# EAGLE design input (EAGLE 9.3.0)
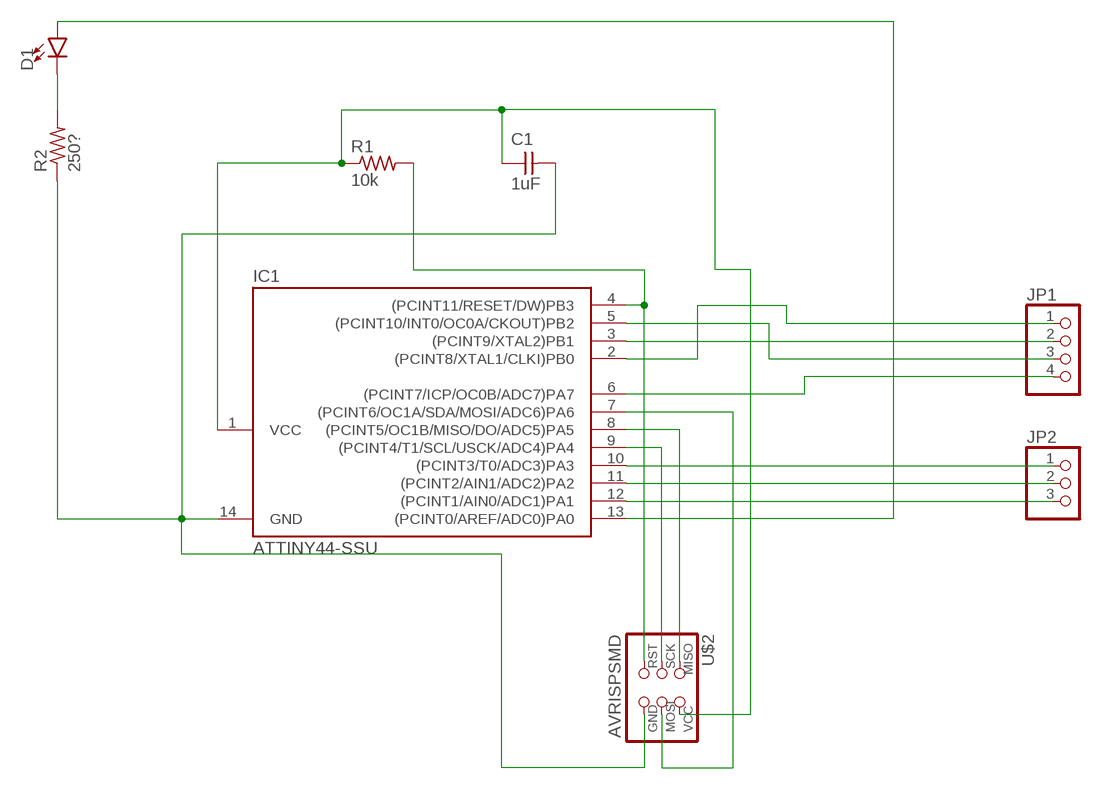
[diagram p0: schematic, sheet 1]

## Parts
C1  1uF  CAP-UNPOLARIZEDFAB  [C1206FAB]
D1  LED1206  [LED-1206]
IC1  ATTINY44-SSU  [SOIC14]
JP1  PINHD-1X41X04_SMT  [1X04_SMT]
JP2  PINHD-1X31X03_SMT  [1X03_SMT]
R1  10k  RES-US1206FAB  [R1206FAB]
R2  250?  RES-US1206FAB  [R1206FAB]
U$2  AVRISPSMD  [2X03SMD]

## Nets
N$1: C1.1 IC1.1(VCC) R1.1 U$2.2(VCC)
N$2: IC1.5((PCINT10/INT0/OC0A/CKOUT)PB2) JP1.3
N$3: C1.2 IC1.14(GND) R2.1 U$2.6(GND)
N$4: IC1.3((PCINT9/XTAL2)PB1) JP1.2
N$5: IC1.8((PCINT5/OC1B/MISO/DO/ADC5)PA5) U$2.1(MISO)
N$6: IC1.9((PCINT4/T1/SCL/USCK/ADC4)PA4) U$2.3(SCK)
N$7: IC1.4((PCINT11/RESET/DW)PB3) R1.2 U$2.5(RST)
N$8: IC1.2((PCINT8/XTAL1/CLKI)PB0) JP1.1
N$9: D1.C R2.2
N$10: IC1.7((PCINT6/OC1A/SDA/MOSI/ADC6)PA6) U$2.4(MOSI)
N$11: D1.A IC1.13((PCINT0/AREF/ADC0)PA0)
N$12: IC1.12((PCINT1/AIN0/ADC1)PA1) JP2.3
N$13: IC1.11((PCINT2/AIN1/ADC2)PA2) JP2.2
N$14: IC1.10((PCINT3/T0/ADC3)PA3) JP2.1
N$15: IC1.6((PCINT7/ICP/OC0B/ADC7)PA7) JP1.4

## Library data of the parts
C1 = fab:CAP-UNPOLARIZED
D1 = SparkFun-LED:LED: LED (Generic)
IC1 = fab:ATTINY44
JP1 = pinhead+:PINHD-1X4: PIN HEADER
JP2 = pinhead+:PINHD-1X3: PIN HEADER
R1 R2 = fab:RES-US: Resistor (US Symbol)
U$2 = fab:AVRISP

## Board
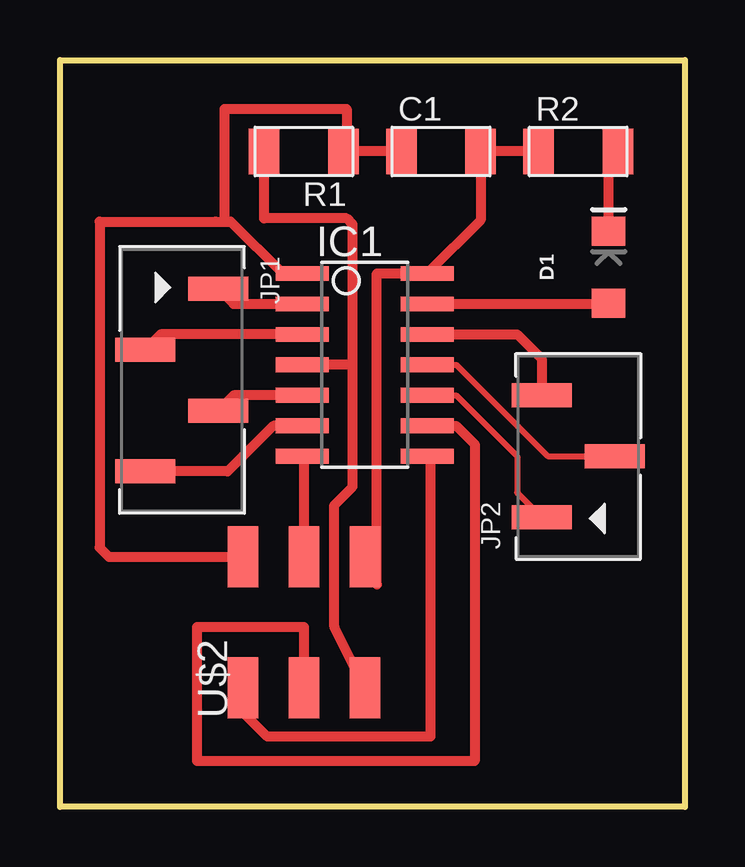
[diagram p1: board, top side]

Size 26.03 x 31.12 mm. Coordinates in mm from the lower left corner, seen from the top.
Outline: 0,31.12 26.03,31.12 26.03,0 0,0 0,31.12
Copper layers (1*16): Top 0.035mm / dielectric 1.5mm / Bottom 0.035mm
Design rules "default": minimum track width 6mil, minimum drill 0.35mm, track to track 6mil, track to pad 6mil, pad to pad 6mil, via to via 6mil, smd to smd 6mil, copper to edge 40mil, drill to drill 6mil, minimum pad ring 10mil, minimum via ring 8mil, stop-mask expansion 4mil, vias tented up to drill 0mil, thermal gap 10mil

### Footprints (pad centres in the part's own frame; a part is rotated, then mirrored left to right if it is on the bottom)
C1206FAB = smd 1.27 x 1.905: 1 -1.651,0; 2 1.651,0
LED-1206 = smd 1.2 x 1.4: A -1.5,0; C 1.5,0
SOIC14 = smd 0.61 x 2.21: 1 -3.81,-2.603; 2 -2.54,-2.603; 3 -1.27,-2.603; 4 0,-2.603; 5 1.27,-2.603; 6 2.54,-2.603; 7 3.81,-2.603; 8 3.81,2.603; 9 2.54,2.603; 10 1.27,2.603; 11 0,2.603; 12 -1.27,2.603; 13 -2.54,2.603; 14 -3.81,2.603
1X04_SMT = smd 1 x 2.5: 1 -3.81,1.52; 2 -1.27,-1.52; 3 1.27,1.52; 4 3.81,-1.52
1X03_SMT = smd 1 x 2.5: 1 -2.54,1.52; 2 0,-1.52; 3 2.54,1.52
R1206FAB = smd 1.27 x 1.905: 1 -1.651,0; 2 1.651,0
2X03SMD = smd 2.54 x 1.27: 1 -2.54,2.54; 2 2.92,2.54; 3 -2.54,0; 4 2.92,0; 5 -2.54,-2.54; 6 2.92,-2.54

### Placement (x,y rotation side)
C1  15.87,27.3 0 top
D1  22.86,22.48 90 top
IC1  12.7,18.41 270 top
JP1  5.08,17.78 270 top
JP2  21.59,14.61 90 top
R1  10.16,27.3 180 top
R2  21.59,27.3 0 top
U$2  10.16,7.49 90 top

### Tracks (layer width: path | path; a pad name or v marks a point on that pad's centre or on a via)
N$1
  Top 0.406: C1.1 R1.1 11.94,27.43 11.94,29.08 6.86,29.08 6.86,24.38 | 6.86,24.38 6.48,24.38 1.65,24.38 1.65,10.8 2.03,10.41 U$2.2 | 6.86,24.38 7.11,24.38 9.27,22.23 IC1.1
N$2
  Top 0.406: IC1.5 7.24,17.14 JP1.3
N$3
  Top 0.406: R2.1 C1.2 17.53,24.45 IC1.14 13.21,22.23 13.21,9.27 U$2.6
N$4
  Top 0.406: JP1.2 4.19,19.69 IC1.3
N$5
  Top 0.406: U$2.1 7.62,3.94 8.64,2.92 15.44,2.92 15.44,14.46 IC1.8
N$6
  Top 0.406: IC1.9 16.51,15.88 17.27,15.11 17.27,1.91 5.71,1.91 5.71,7.49 10.16,7.49 U$2.3
N$7
  Top 0.406: U$2.5 11.43,7.49 11.43,12.57 12.19,13.34 12.19,18.41 | 12.19,18.41 IC1.4 | 12.19,18.41 12.19,24.26 11.94,24.51 8.51,24.51 R1.2
N$8
  Top 0.406: JP1.1 7.24,20.96 IC1.2
N$9
  Top 0.406: D1.C 22.86,26.92 R2.2
N$10
  Top 0.406: IC1.7 10.16,14.54 U$2.4
N$11
  Top 0.406: D1.A 22.86,20.96 IC1.13
N$12
  Top 0.406: IC1.12 19.05,19.69 20.07,18.66 JP2.3
N$13
  Top 0.254: IC1.11 16.51,18.41 20.32,14.61 JP2.2
N$14
  Top 0.254: IC1.10 16.51,17.14 19.05,14.61 19.05,13.09 JP2.1
N$15
  Top 0.406: IC1.6 8.89,15.88 6.99,13.97 JP1.4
